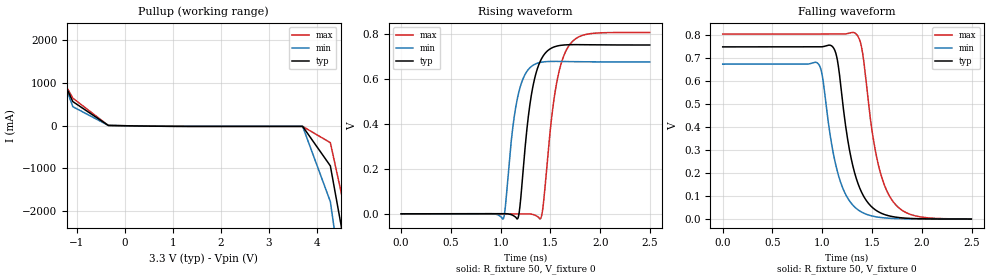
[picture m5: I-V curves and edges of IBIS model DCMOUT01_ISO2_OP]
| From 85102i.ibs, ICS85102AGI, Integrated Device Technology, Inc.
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[Model]   DCMOUT01_ISO2_OP
Model_type   Open_source
Polarity   Non-Inverting
|   typ   min   max
C_comp   2pF   1.5pF   2.5pF
Vmeas = .344V
Rref = 50
Cref = 0
Vref = 0V
|   typ   min   max
[Voltage range]   3.3V   3.135V   3.465V
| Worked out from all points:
|   slope of the pullup table from 0 to 0.495 V, typ, clamps not added: 54.5 ohm
|   rising waveform, R_fixture 50, V_fixture 0: 20-80 % time 123ps typ, 114ps min, 139ps max; typ from 0 V to 0.749 V
|   falling waveform, R_fixture 50, V_fixture 0: 20-80 % time 182ps typ, 179ps min, 184ps max; typ from 0.749 V to 0 V
[Pullup]
|Voltage   I (typ)   I (min)   I (max)
-3.3V     5.929A     7.281A     5.128A
-2.56V    4.138A     5A         3.631A
-1.82V    2.349A     2.722A     2.136A
-1.08V    565.7mA    446.7mA    647.1mA
-340mV    7.268mA    8.174mA    6.641mA
3.71V     -15.08mA   -14.13mA   -16.17mA
4.288V    -939.9mA   -1.778A    -395.8mA
4.866V    -4.531A    -6.361A    -3.386A
6.6V      -15.32A    -20.11A    -12.39A
[Ramp]
|   typ   min   max
dV/dt_r   0.618/0.195n   0.559/0.181n   0.661/0.221n
dV/dt_f   0.605/0.294n   0.545/0.287n   0.649/0.3n
R_load =   50.0000
[Rising Waveform]
R_fixture = 50
V_fixture = 0
V_fixture_max = 0
V_fixture_min = 0
C_fixture = 0.0p
| Time   typ   min   max
0s        1.469nV    329.3pV    95.28nV
1.026ns   401.4uV    -22.55mV   617.5nV
1.119ns   -5.95mV    370.6mV    -10.36uV
1.171ns   -21.47mV   518.2mV    2.251uV
1.294ns   484.8mV    647.9mV    -448.4uV
1.399ns   677.8mV    671.8mV    -22.17mV
1.429ns   701.6mV    674mV      42.96mV
1.547ns   741.9mV    676.3mV    539.5mV
1.672ns   750mV      675.5mV    736mV
2.498ns   748.9mV    673.8mV    804.6mV
[Falling Waveform]
R_fixture = 50
V_fixture = 0
V_fixture_max = 0
V_fixture_min = 0
C_fixture = 0.0p
| Time   typ   min   max
0s        748.9mV    673.8mV    804.6mV
953.5ps   748.5mV    678.1mV    804.6mV
1.001ns   749.6mV    621.8mV    804.6mV
1.101ns   750.8mV    308.7mV    804.7mV
1.154ns   687.2mV    203.9mV    804.5mV
1.334ns   187.9mV    49.06mV    807.6mV
1.401ns   111mV      28.85mV    732.3mV
1.549ns   35.42mV    9.066mV    263.9mV
1.689ns   12.05mV    3.027mV    89.91mV
2.498ns   24.47uV    5.43uV     200.3uV
